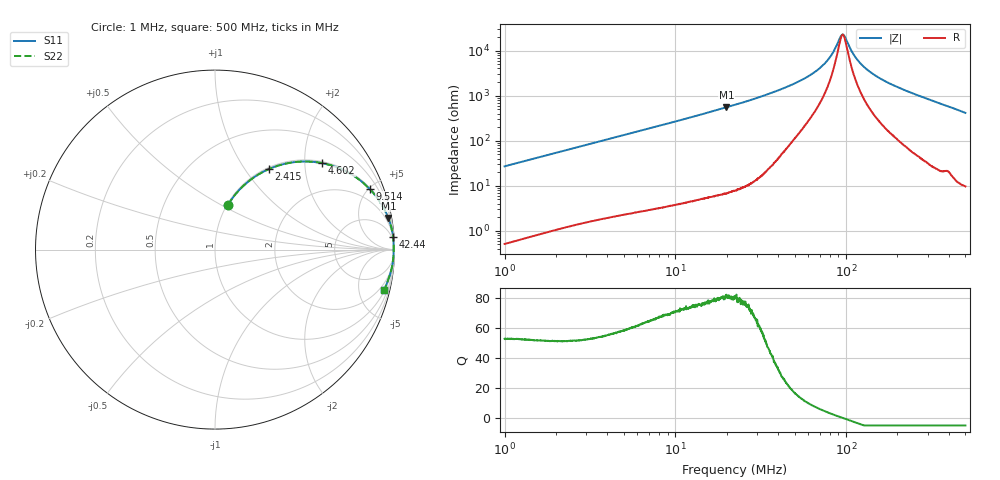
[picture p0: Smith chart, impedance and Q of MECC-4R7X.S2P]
!s-Parameter Generated by FASTRON Sdn. Bhd.
!FASTRON P/N : MECC-4R7X
!Keysight Technologies,E4991B,MY54100416,A.01.15
!Date: Thu Apr 02 10:01:12 2026
!Version  : Rev00 Thu Apr 02 10:01:12 2026
!Data & Calibration Information:
!PortZ  Port1:50+j0  Port2:50+j0
!When reading, reference impedance value at option line is always used.
!Remarks : This data is being provided solely for informational purposes.
!Freq	S11	S21	S12	S22
# Hz S dB R 50
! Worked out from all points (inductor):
!   1601 points, 1 MHz to 500 MHz, reference 50 ohm
!   read as one part in series: L = 4.29 uH near 1.032 MHz
!   highest Q = 80.8 at 19.9 MHz (marker M1), where L = 4.38 uH
!   self-resonance near 95.58 MHz
!   S11 on the Smith chart (normalised r, x): 1 MHz: 1.01, +0.54; 2.415 MHz: 1.03, +1.29; 4.602 MHz: 1.04, +2.45; 9.514 MHz: 1.07, +5.07; 42.44 MHz: 2, +28; 500 MHz: 1.19, -8.28
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1000000  -11.71 73.9  -0.35 -15.1  -0.35 -15.1  -11.71 73.9
1575296  -8.23 66.1  -0.78 -22.8  -0.78 -22.8  -8.23 66.1
2414996  -5.38 56.3  -1.59 -32.6  -1.59 -32.6  -5.38 56.3
2820919  -4.49 52.3  -2.03 -36.6  -2.03 -36.6  -4.49 52.3
4601872  -2.30 38.9  -4.05 -50.1  -4.05 -50.1  -2.30 38.9
7957584  -0.93 25.1  -7.43 -64.0  -7.43 -64.0  -0.93 25.1
9514295  -0.67 21.4  -8.74 -67.7  -8.74 -67.7  -0.67 21.4
1.99012e7  -0.16 10.3  -14.94 -79.0  -14.94 -79.0  -0.16 10.3
2.236068e7  -0.13 9.1  -16.03 -80.2  -16.03 -80.2  -0.13 9.1
4.2444e7  -0.04 4.0  -23.12 -83.9  -23.12 -83.9  -0.04 4.0
6.307767e7  -0.04 1.9  -29.62 -81.3  -29.62 -81.3  -0.04 1.9
7.81003e7  -0.04 0.9  -35.79 -73.9  -35.79 -73.9  -0.04 0.9
8.440921e7  -0.04 0.6  -39.53 -65.3  -39.53 -65.3  -0.04 0.6
9.265618e7  -0.04 0.1  -46.00 -28.8  -46.00 -28.8  -0.04 0.1
9.595246e7  -0.04 -0.0  -47.11 3.2  -47.11 3.2  -0.04 -0.0
9.89808e7  -0.04 -0.2  -45.78 31.0  -45.78 31.0  -0.04 -0.2
1.107821e8  -0.04 -0.7  -38.25 68.2  -38.25 68.2  -0.04 -0.7
1.230311e8  -0.04 -1.1  -33.90 76.2  -33.90 76.2  -0.04 -1.1
1.437107e8  -0.04 -1.9  -29.63 80.4  -29.63 80.4  -0.04 -1.9
1.77937e8  -0.05 -3.0  -25.61 82.2  -25.61 82.2  -0.05 -3.0
2.563485e8  -0.08 -5.4  -20.53 82.0  -20.53 82.0  -0.08 -5.4
5e8  -0.29 -13.5  -12.63 75.2  -12.63 75.2  -0.29 -13.5
